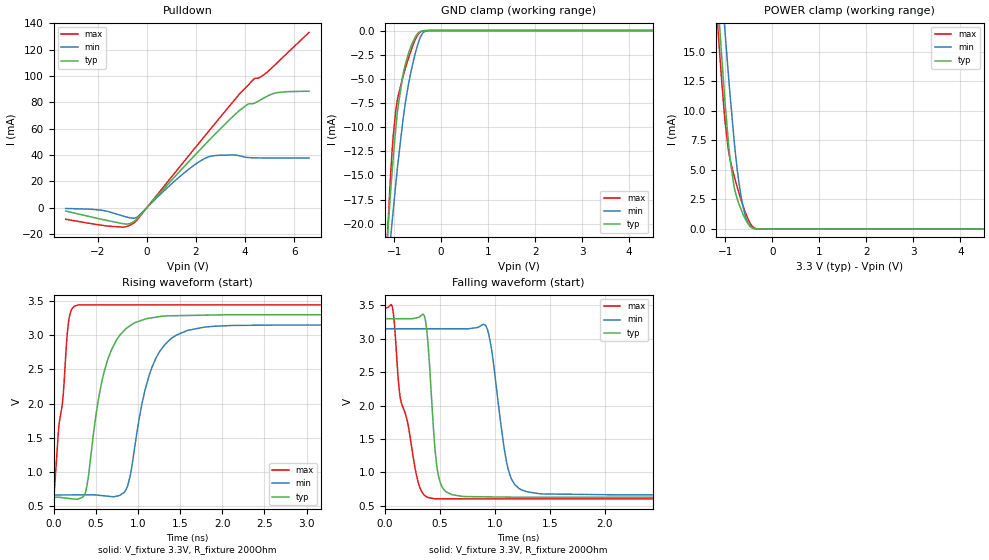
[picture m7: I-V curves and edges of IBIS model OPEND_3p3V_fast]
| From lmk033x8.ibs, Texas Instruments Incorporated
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[Model]   OPEND_3p3V_fast
Model_type   Open_drain
Polarity   Non-Inverting
Vmeas = 1.65
Vref = 3.3
Cref = 15pF
Rref = 200
|   typ   min   max
|   (nom PVT)   (fast PVT)   (slow PVT)
C_comp   0.571p   0.551p   0.636p
|C_comp (ON state)   0.733p   0.694p   0.771p
|C_comp (OFF state)   0.571p   0.551p   0.636p
[Voltage Range]   3.3   3.15   3.45
[Temperature Range]   27   125   -40
[Pullup Reference]   3.3   3.15   3.45
[Pulldown Reference]   0   0   -0
[Power Clamp Reference]   3.3   3.15   3.45
[GND Clamp Reference]   0   0   0
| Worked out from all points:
|   slope of the pulldown table from 0 to 0.495 V, typ, clamps not added: 48 ohm
|   GND clamp passes 1 mA (typ) near -0.58 V on its own axis
|   POWER clamp passes 1 mA (typ) near -0.60 V on its own axis
|   falling waveform, V_fixture 3.3V, R_fixture 200Ohm: 20-80 % time 68.2ps typ, 120ps min, 162ps max; typ from 3.3 V to 0.629 V
|   rising waveform, V_fixture 3.3V, R_fixture 200Ohm: 20-80 % time 244ps typ, 271ps min, 119ps max; typ from 0.63 V to 3.3 V
[Pulldown]
|   Voltage   I(typ)   I(min)   I(max)
-3.3V     -2.52mA    -600.3uA   -8.758mA
-1.865V   -8.706mA   -1.855mA   -13.25mA
-963.6mV  -12.15mA   -6.33mA    -14.77mA
-528mV    -10.55mA   -7.967mA   -11.61mA
-379.5mV  -7.92mA    -6.939mA   -8.819mA
1.541V    31.66mA    26.77mA    35.73mA
2.511V    50.79mA    38.65mA    57.96mA
3.482V    68.92mA    40.03mA    79.92mA
4.125V    78.74mA    38.11mA    93.15mA
4.372V    79.36mA    37.88mA    97.98mA
5.273V    87.34mA    37.74mA    109.6mA
6.6V      88.5mA     37.75mA    133.2mA
[GND Clamp]
|   Voltage   I(typ)   I(min)   I(max)
-3.3V     -203.8mA   -156.3mA   -307mA
-1.171V   -23.41mA   -26.67mA   -23.99mA
-1.073V   -16.48mA   -21.32mA   -14.64mA
-1.053V   -15.2mA    -20.29mA   -13.1mA
-1.023V   -13.35mA   -18.76mA   -11.08mA
-963.6mV  -10.02mA   -15.81mA   -8.174mA
-924mV    -8.154mA   -13.94mA   -6.971mA
-815.1mV  -4.636mA   -9.357mA   -4.815mA
-636.9mV  -1.582mA   -4.164mA   -2.006mA
-438.9mV  -95.08uA   -660.3uA   -145.6uA
-260.7mV  -658.8nA   -9.216uA   -902.5nA
6.6V      0A         0A         0A
[POWER Clamp]
|   Voltage   I(typ)   I(min)   I(max)
-3.3V     163.1mA    154.7mA    175.2mA
-1.162V   19.42mA    25.01mA    17.09mA
-1.092V   15.36mA    21.2mA     13.24mA
-1.013V   11.02mA    16.97mA    9.368mA
-933.9mV  7.229mA    12.94mA    6.584mA
-904.2mV  6.039mA    11.5mA     5.927mA
-815.1mV  3.558mA    7.522mA    4.491mA
-716.1mV  2.165mA    4.038mA    3.108mA
-656.7mV  1.543mA    2.548mA    2.342mA
-567.6mV  770.8uA    1.019mA    1.318mA
-409.2mV  60.75uA    64.51uA    154.9uA
6.6V      0A         0A         0A
[Ramp]
R_load = 200
|   typ   min   max
dV/dt_r   1.60189/2.43817e-10   1.49103/2.71112e-10   1.70661/1.18896e-10
dV/dt_f   1.60248/6.77366e-11   1.49103/1.19833e-10   1.71296/1.61621e-10
[Falling Waveform]
V_fixture = 3.3V
V_fixture_min = 3.15V
V_fixture_max = 3.45V
R_fixture = 200Ohm
C_fixture = 0F
|   Time   V(typ)   V(min)   V(max)
0s        3.3V       3.15V      3.453V
70.66ps   3.3V       3.15V      3.463V
142.1ps   3.3V       3.15V      2.105V
358.6ps   3.345V     3.15V      661.8mV
456.2ps   1.346V     3.15V      605.7mV
549.5ps   721mV      3.15V      605.7mV
918.8ps   635.5mV    3.191V     605.5mV
1.135ns   631mV      966.1mV    605.4mV
1.405ns   629.4mV    682.3mV    605.3mV
19ns      629.2mV    665mV      598.3mV
[Rising Waveform]
V_fixture = 3.3V
V_fixture_min = 3.15V
V_fixture_max = 3.45V
R_fixture = 200Ohm
C_fixture = 0F
|   Time   V(typ)   V(min)   V(max)
0s        630.2mV    665mV      605.6mV
177.1ps   615.6mV    666mV      3.186V
293.2ps   607.7mV    666.7mV    3.444V
394.4ps   787.5mV    667.3mV    3.444V
599.8ps   2.464V     652.8mV    3.444V
861.9ps   3.101V     748mV      3.444V
1.087ns   3.237V     2.211V     3.444V
1.279ns   3.277V     2.798V     3.444V
2.119ns   3.3V       3.143V     3.444V
19ns      3.3V       3.15V      3.45V
